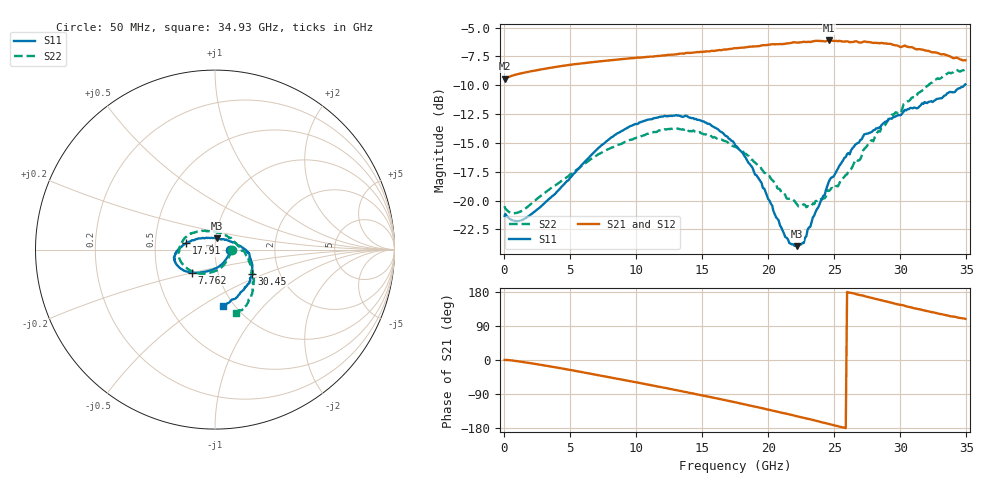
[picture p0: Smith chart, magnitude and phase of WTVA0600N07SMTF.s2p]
! 50 ohm 2-Port S-parameters measured by Modelithics Inc support@modelithics.com  Tampa, FL USA 813-866-6335 (February 2024)
! Smiths Interconnect,  6dB P/N: WTVA0600N07SMTF, Temperature: -25 C
! Board: 10 mil Rogers 4350B, Mounting Pad Dimensions: Length: 15 mils, Width: 25 mils, Gap: 40 mils.
# Hz S RI R 50
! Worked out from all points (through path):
!   352 points, 50 MHz to 34.93 GHz, reference 50 ohm
!   highest |S21| = -6.11 dB at 24.58 GHz (marker M1); lowest = -9.4 dB at 50 MHz (marker M2)
!   group delay of S21, straight-line fit = 20.7 ps
!   lowest |S11| = -24.0 dB at 22.19 GHz (marker M3), VSWR 1.14, Z = 50.9 + j6.34 ohm
!   |S11| at or under -10 dB: start of sweep to 34.85 GHz
!   |S22| runs from -21.1 to -8.6 dB; largest |S21 - S12| = 0.0047
!   S11 on the Smith chart (normalised r, x): 50 MHz: 1.19, -0.01; 7.762 GHz: 0.75, -0.20; 17.91 GHz: 0.72, +0.05; 30.45 GHz: 1.45, -0.41; 34.93 GHz: 0.89, -0.62
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5e7  0.0858 -0.00325  0.3373 0.00137  0.337 0.000908  0.0944 -0.00322
6.975e8  0.0738 -0.0354  0.3489 -0.00996  0.3485 -0.01  0.0795 -0.0379
1.792e9  0.0513 -0.0677  0.3584 -0.0451  0.3579 -0.0452  0.0583 -0.0737
5.8715e9  -0.067 -0.1255  0.3346 -0.2065  0.334 -0.2066  -0.0481 -0.1326
7.762e9  -0.1273 -0.1284  0.2911 -0.2805  0.2904 -0.2804  -0.1012 -0.1313
1.1742e10  -0.215 -0.0827  0.1411 -0.3994  0.1397 -0.3994  -0.1881 -0.0718
1.5125e10  -0.2194 -0.0195  -0.0334 -0.4412  -0.0348 -0.4406  -0.1926 0.0209
1.7513e10  -0.1709 0.0288  -0.1696 -0.4249  -0.1709 -0.4238  -0.1531 0.0765
1.7911e10  -0.1604 0.0351  -0.1925 -0.4176  -0.1939 -0.4163  -0.1437 0.0842
1.9503e10  -0.1032 0.0595  -0.2818 -0.3771  -0.2826 -0.3758  -0.0916 0.1015
2.1294e10  -0.0262 0.0643  -0.3721 -0.3008  -0.3729 -0.2989  -0.0261 0.1023
2.21895e10  0.0132 0.062  -0.413 -0.2523  -0.4135 -0.2501  0.00877 0.0958
2.2687e10  0.033 0.0564  -0.4331 -0.2245  -0.4332 -0.2226  0.0255 0.0929
2.33835e10  0.0649 0.0542  -0.4554 -0.1828  -0.4554 -0.181  0.0509 0.0827
2.45775e10  0.1143 0.037  -0.4848 -0.0983  -0.4846 -0.0963  0.0935 0.0579
2.5274e10  0.1354 0.0225  -0.4886 -0.0455  -0.488 -0.0437  0.1084 0.0386
2.7264e10  0.192 -0.0247  -0.4809 0.0933  -0.4797 0.0953  0.1665 -0.0155
2.91545e10  0.2083 -0.0875  -0.4248 0.2201  -0.423 0.2219  0.2075 -0.0955
3.005e10  0.2044 -0.1155  -0.3803 0.2636  -0.3785 0.2651  0.2036 -0.1291
3.0448e10  0.2066 -0.1336  -0.3659 0.2887  -0.3636 0.2905  0.2155 -0.1555
3.2637e10  0.1637 -0.2179  -0.2489 0.3618  -0.2472 0.3621  0.1995 -0.2672
3.49255e10  0.0448 -0.3157  -0.1291 0.3848  -0.1253 0.3854  0.1162 -0.3518
